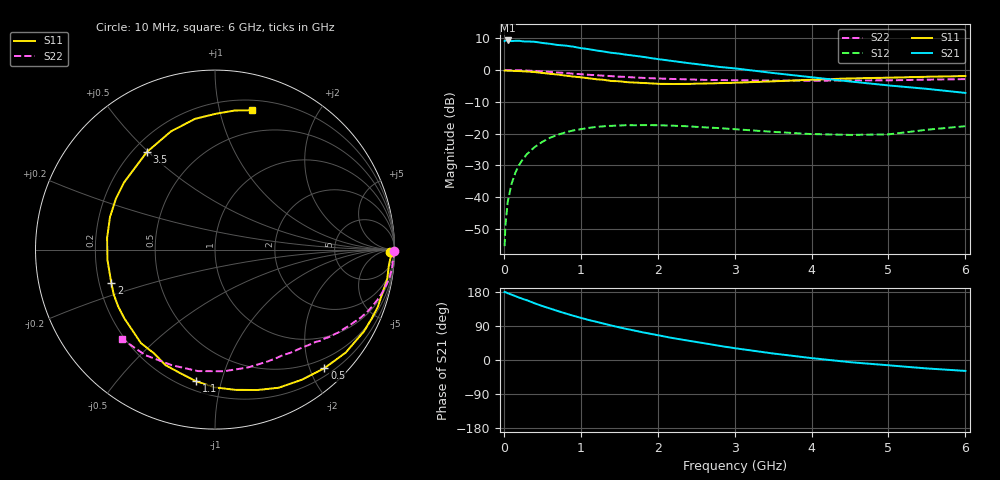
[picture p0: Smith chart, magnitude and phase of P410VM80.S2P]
! SIEMENS Small Signal Semiconductors
! BFP182
! Si NPN RF Bipolar Junction Transistor in SOT143
! VCE = 10 V  IC = 0.8 mA
! Common Emitter S-Parameters:  March  1996
# GHz  S  MA  R  50
!  f  S11  S21  S12  S22
! GHz  MAG  ANG  MAG  ANG  MAG  ANG  MAG  ANG
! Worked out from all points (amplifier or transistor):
!   36 points, 10 MHz to 6 GHz, reference 50 ohm
!   highest |S21| = 9.3 dB at 50 MHz (marker M1)
!   |S21| within 3 dB of that: start of sweep to 1.168 GHz
!   unconditionally stable (mu >= 1): 2.771 GHz to end of sweep
!   at 250 MHz: K = 0.09, MSG = 18.5 dB, |S12| = -28.0 dB
!   at 1.4 GHz: K = 0.52, MSG = 11.5 dB, |S12| = -17.5 dB
!   at 6 GHz: K = 1.14, MAG = 3.0 dB, |S12| = -17.7 dB
!   S11 on the Smith chart (normalised r, x): 10 MHz: 57, -36; 500 MHz: 0.33, -2.24; 1.1 GHz: 0.26, -0.83; 2 GHz: 0.25, -0.15; 3.5 GHz: 0.25, +0.49; 6 GHz: 0.29, +1.26
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0.01  0.9751 -0.9  2.852 179.5  0.0017 89.7  0.9972 -0.3
0.02  0.981 -2.2  2.908 179.0  0.0035 85.2  0.9962 -0.7
0.05  0.973 -4.8  2.912 176.3  0.0084 88.1  0.9969 -1.8
0.1  0.9734 -9.6  2.847 172.4  0.0162 83.7  0.9928 -3.5
0.2  0.9616 -19.5  2.878 164.6  0.0324 77.5  0.9893 -7.1
0.4  0.9273 -38.2  2.777 149.6  0.0614 65.9  0.9654 -13.8
0.5  0.8989 -47.3  2.661 142.4  0.0742 60.1  0.9491 -16.9
0.6  0.8719 -56.2  2.579 135.9  0.0859 54.7  0.932 -19.8
0.8  0.8169 -73.3  2.418 123.0  0.1044 44.8  0.8952 -25.1
0.9  0.7891 -81.9  2.328 117.0  0.1119 40.6  0.8752 -27.4
1.1  0.7412 -98.1  2.129 105.8  0.123 32.4  0.8411 -31.8
1.5  0.6646 -128.4  1.807 86.2  0.1341 19.3  0.7859 -39.1
1.8  0.6257 -149.5  1.615 73.3  0.1357 12.0  0.7524 -44.0
2  0.6066 -162.4  1.485 65.5  0.1355 7.6  0.7364 -47.1
2.2  0.6022 -174.9  1.381 57.7  0.1332 4.0  0.7224 -50.5
2.6  0.6125 162.8  1.2 44.4  0.1256 -1.4  0.6993 -57.1
3  0.63 143.7  1.061 31.2  0.1173 -5.3  0.6892 -64.5
3.5  0.6633 124.9  0.897 17.2  0.1066 -6.1  0.6819 -74.4
4  0.7026 110.5  0.769 5.0  0.0983 -2.8  0.6796 -85.7
4.5  0.7369 98.7  0.66 -5.7  0.0955 2.2  0.6835 -98.0
5.5  0.7828 81.9  0.505 -22.3  0.115 14.9  0.7048 -123.5
6  0.803 75.2  0.436 -28.8  0.1308 14.8  0.7188 -136.2
